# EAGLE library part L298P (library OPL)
DUAL FULL-BRIDGE DRIVER
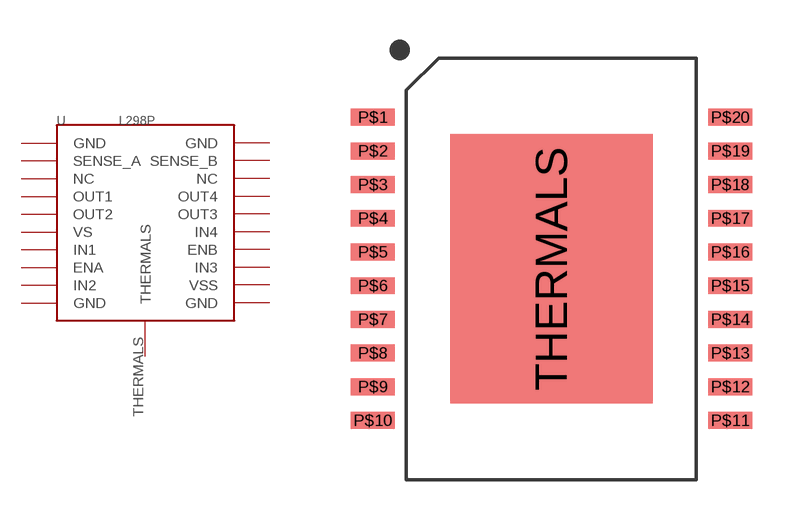
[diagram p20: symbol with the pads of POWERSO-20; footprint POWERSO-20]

Designator prefix U

## L298P-310040018  [POWERSO-20]
P$1  GND
P$2  SENSE_A
P$3  NC
P$4  OUT1
P$5  OUT2
P$6  VS
P$7  IN1
P$8  ENA
P$9  IN2
P$10  GND
P$11  GND
P$12  VSS
P$13  IN3
P$14  ENB
P$15  IN4
P$16  OUT3
P$17  OUT4
P$18  NC
P$19  SENSE_B
P$20  GND
THERMALS  THERMALS

## Footprint POWERSO-20 (pad centres in mm)
smd 1.651 x 0.635: P$1 -6.731,5.715; P$2 -6.731,4.445; P$3 -6.731,3.175; P$4 -6.731,1.905; P$5 -6.731,0.635; P$6 -6.731,-0.635; P$7 -6.731,-1.905; P$8 -6.731,-3.175; P$9 -6.731,-4.445; P$10 -6.731,-5.715; P$11 6.731,-5.715; P$12 6.731,-4.445; P$13 6.731,-3.175; P$14 6.731,-1.905; P$15 6.731,-0.635; P$16 6.731,0.635; P$17 6.731,1.905; P$18 6.731,3.175; P$19 6.731,4.445; P$20 6.731,5.715
smd 7.62 x 10.16: THERMALS 0,0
